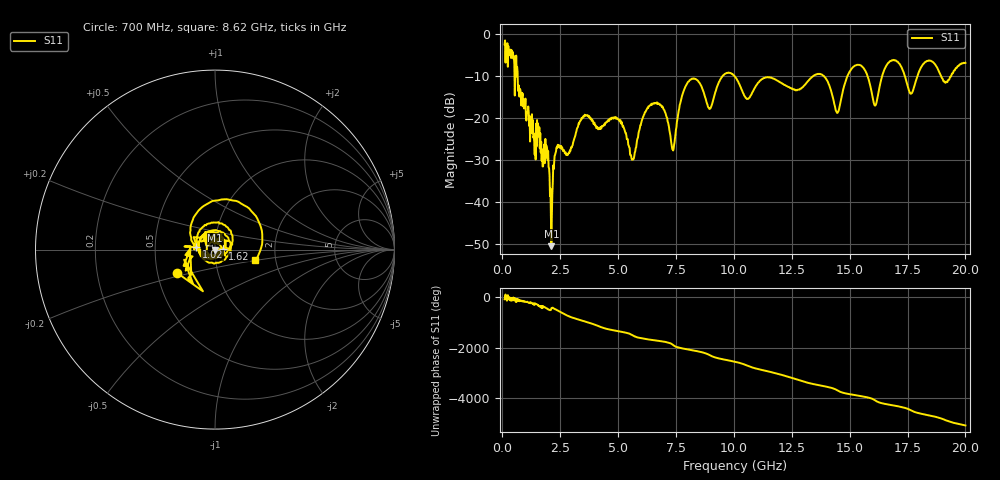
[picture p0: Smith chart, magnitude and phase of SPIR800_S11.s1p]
!Keysight Technologies,P9374A,MY57211922,A.15.40.13
!Date: Friday, October 24, 2025 11:24:55
!Correction: S11(C  1-Port  )
!S1P File: Measurement: S11:
# Hz S  dB  R 50
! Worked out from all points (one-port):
!   996 points, 100 MHz to 20 GHz, reference 50 ohm
!   lowest |S11| = -50.6 dB at 2.12 GHz (marker M1), VSWR 1.01, Z = 50.1 - j0.288 ohm
!   |S11| at or under -10 dB: 664.9 MHz to 9.507 GHz (8.842 GHz wide, 174 % of centre); 10.04 GHz to 13.42 GHz (3.381 GHz wide, 28.8 % of centre); 13.9 GHz to 14.9 GHz (1.004 GHz wide, 6.98 % of centre)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
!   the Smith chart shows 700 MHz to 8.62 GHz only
!   S11 on the Smith chart (normalised r, x): 700 MHz: 0.63, -0.18; 1.02 GHz: 0.81, +0.02; 1.62 GHz: 1.09, +0.01; 8.62 GHz: 1.56, -0.20
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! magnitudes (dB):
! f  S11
! 100 MHz  -2.4
! 700 MHz  -12.1
! 1.02 GHz  -19.6
! 1.62 GHz  -27.2
! 1.94 GHz  -27.5
! 2.12 GHz  -50.6
! 2.32 GHz  -28.0
! 2.6 GHz  -27.2
! 3.56 GHz  -19.2
! 5.08 GHz  -20.8
! 5.62 GHz  -29.9
! 6.36 GHz  -17.1
! 6.94 GHz  -17.5
! 7.36 GHz  -27.5
! 7.58 GHz  -19.6
! 8.04 GHz  -11.3
! 8.62 GHz  -12.7
! 8.96 GHz  -17.8
! 10.06 GHz  -10.2
! 12.54 GHz  -13.0
! 13.8 GHz  -9.6
! 14.48 GHz  -18.7
! 15.04 GHz  -8.5
! 15.6 GHz  -8.0
! 16.1 GHz  -17.0
! 16.8 GHz  -6.3
! 17.52 GHz  -12.6
! 20 GHz  -6.8
